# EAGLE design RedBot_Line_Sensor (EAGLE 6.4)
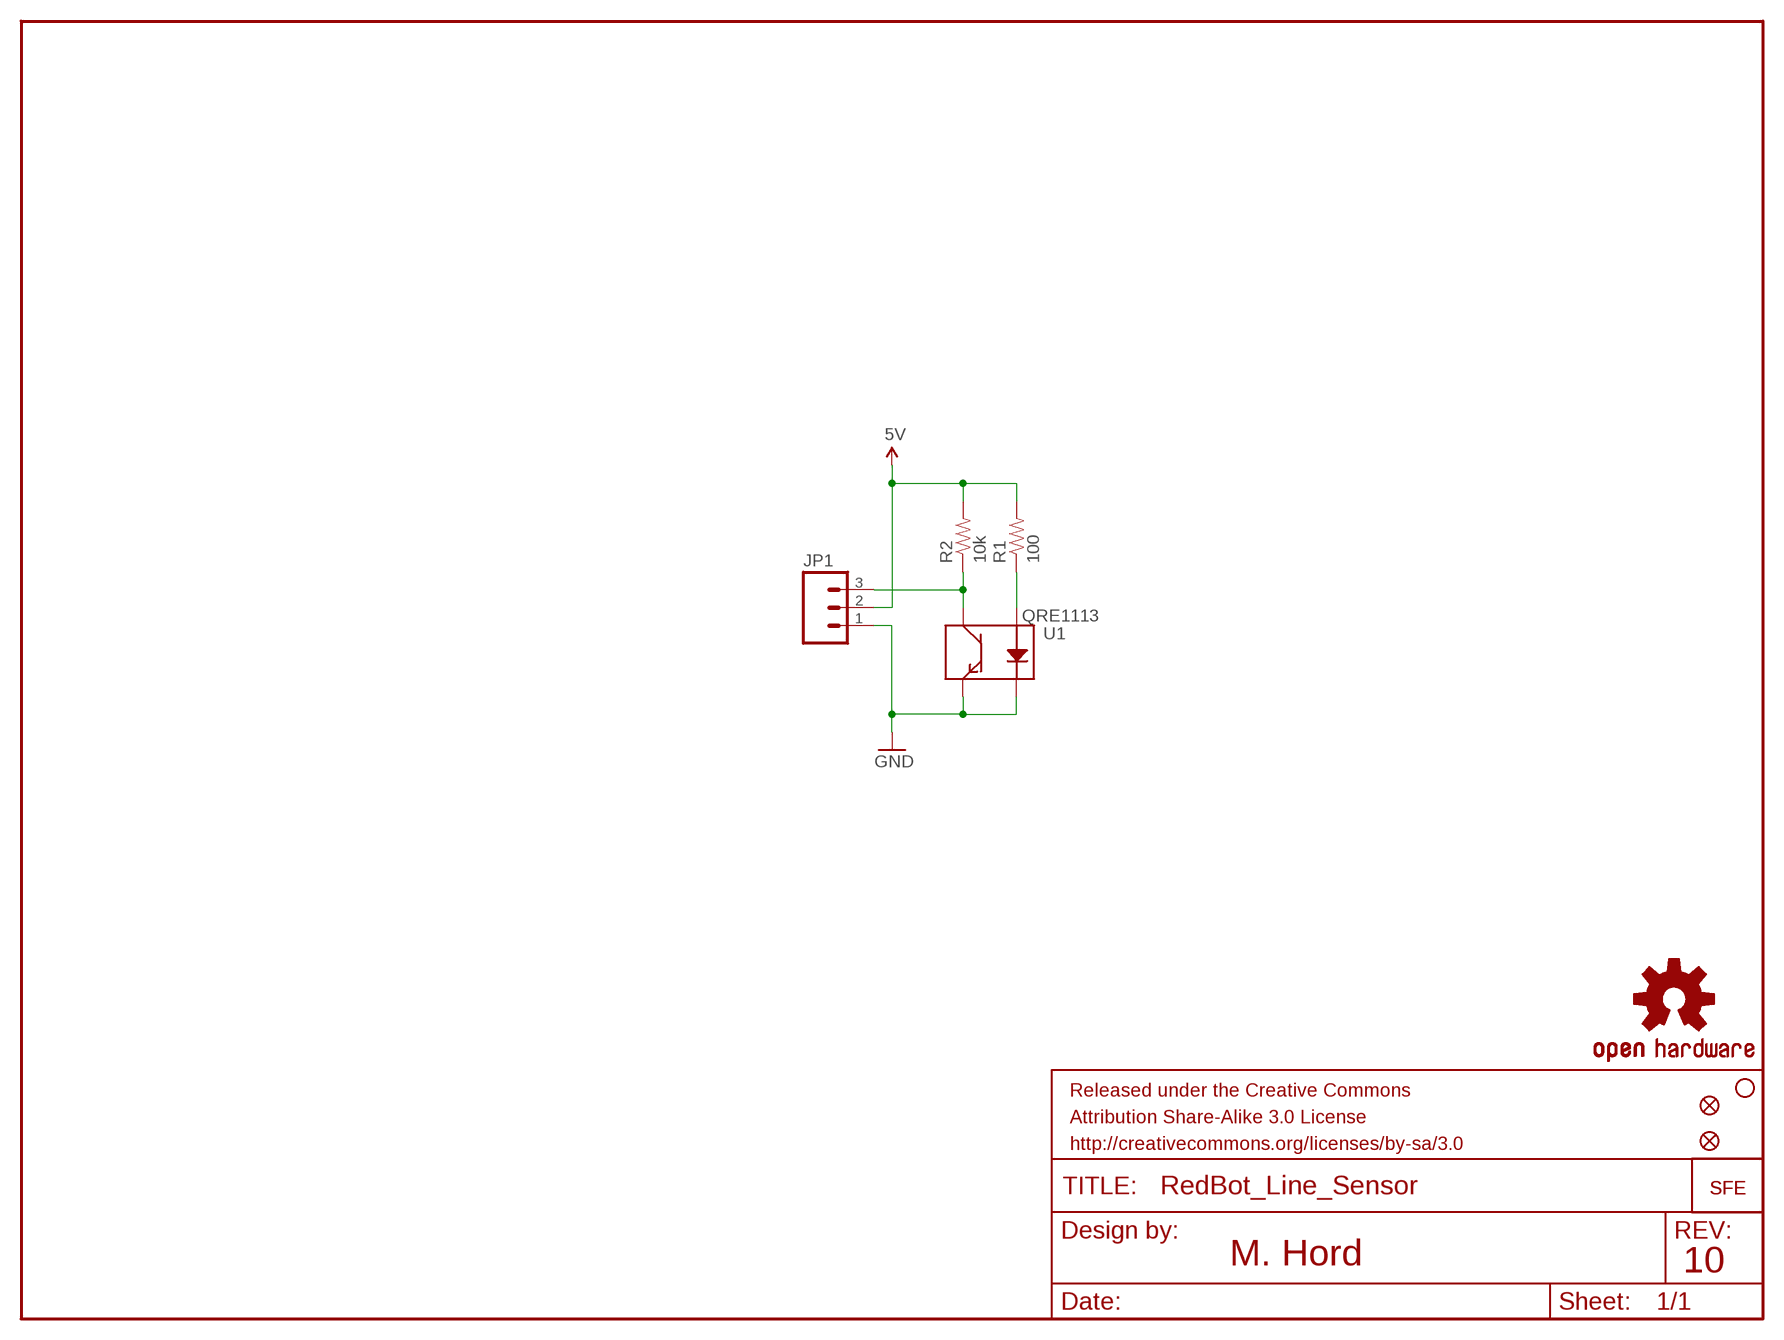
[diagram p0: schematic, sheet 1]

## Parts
FID1  FIDUCIALUFIDUCIAL  [MICRO-FIDUCIAL]
FID2  FIDUCIALUFIDUCIAL  [MICRO-FIDUCIAL]
FRAME1  FRAME-LETTER  [CREATIVE_COMMONS]
JP1  M03SMD_RA_MALE  [1X03_SMD_RA_MALE]
LOGO1  LOGO-SFESK  [SFE-LOGO-FLAME]
LOGO2  OSHW-LOGOS  [OSHW-LOGO-S]
LOGO3  LOGO-SFESK  [SFE-LOGO-FLAME]
R1  100  100-1%  [0402-RES]
R2  10k  10KOHM1/10W1%(0603)  [0402-RES]
STANDOFF1  STAND-OFF  [STAND-OFF]
U1  QRE1113  [QRE1113]

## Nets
5V: JP1.2 R1.2 R2.2
GND: JP1.1 U1.2(K) U1.4(E)
N$1: R1.1 U1.1(A)
N$2: JP1.3 R2.1 U1.3(C)

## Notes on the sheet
- M. Hord | 10

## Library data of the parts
FID1 FID2 = SparkFun-Aesthetics:FIDUCIAL: Fiducial Alignment Points
FRAME1 = SparkFun-Aesthetics:FRAME-LETTER: Schematic Frame
JP1 = SparkFun-Connectors:M03: Header 3 Standard 3-pin 0.1" header. Use with straight break away headers (SKU : PRT-00116), right angle break away headers (PRT-00553), swiss pins (PRT-00743), machine pins (PRT-00117), and female headers (PRT-00115). Molex polarized connector foot print use with SKU : PRT-08232 with associated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; PROD_ID: CONN-10925
LOGO1 LOGO3 = SparkFun-Aesthetics:LOGO-SFE: Spark Fun Electronics PCB Logo
LOGO2 = SparkFun-Aesthetics:OSHW-LOGO: Open Source Hardware Logo This logo indicates the piece of hardware it is found on incorporates a OSHW license and/or adheres to the definition of open source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
R1 = SparkFun-Resistors:100-1%: 100-ohm SMT; PROD_ID: RES-07863
R2 = SparkFun-Resistors:10KOHM1/10W1%(0603): RES-00824; PROD_ID: RES-00824
STANDOFF1 = SparkFun-Electromechanical:STAND-OFF: #4 Stand Off
U1 = SparkFun-Sensors:QRE1113: Reflective object sensor; PROD_ID: IC-09357

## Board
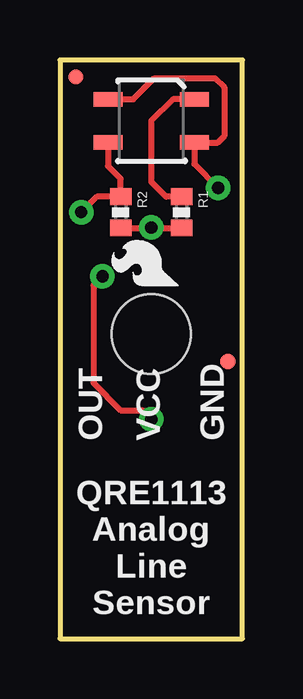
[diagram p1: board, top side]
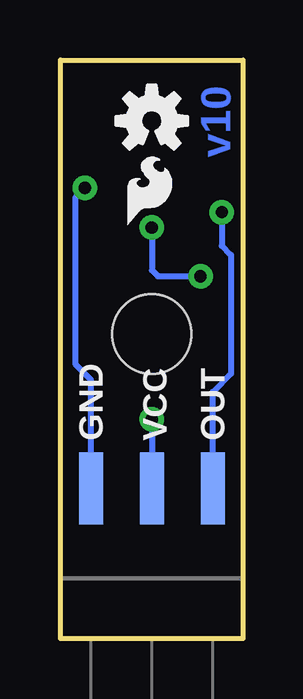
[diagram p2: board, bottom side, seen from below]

Size 7.62 x 24.13 mm. Coordinates in mm from the lower left corner, seen from the top.
Outline: 0,0 7.62,0 7.62,24.13 0,24.13 0,0
Copper layers (1*16): Top 0.035mm / dielectric 1.5mm / Bottom 0.035mm
Design rules "Sparkfun": minimum track width 8mil, minimum drill 20mil, track to track 8mil, track to pad 8mil, pad to pad 8mil, via to via 8mil, smd to smd 8mil, copper to edge 8mil, drill to drill 8mil, minimum pad ring 12mil, minimum via ring 10mil, stop-mask expansion 4mil, vias tented up to drill 20mil, thermal gap 10mil

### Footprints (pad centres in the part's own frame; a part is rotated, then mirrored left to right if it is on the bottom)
MICRO-FIDUCIAL = smd 0.635 x 0.635: 1 0,0
1X03_SMD_RA_MALE = smd 1 x 3: 1 -2.54,5; 2 0,5; 3 2.54,5
0402-RES = smd 0.7 x 0.9: 1 -0.65,0; 2 0.65,0
STAND-OFF = hole 3.302: 0,0
QRE1113 = smd 1.2 x 0.6: 1 -1.8,-0.9; 2 1.8,-0.9; 3 1.8,0.9; 4 -1.8,0.9

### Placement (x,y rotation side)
FID1  7.01,11.56 0 top
FID2  0.66,23.42 0 top
FRAME1  not placed on the board
JP1  3.81,1.27 0 bottom
LOGO1  4.95,14.73 90 top
LOGO2  3.81,21.59 0 bottom
LOGO3  4.83,17.27 0 bottom
R1  5.08,17.78 270 top
R2  2.54,17.78 270 top
STANDOFF1  3.81,12.7 0 top
U1  3.81,21.59 180 top

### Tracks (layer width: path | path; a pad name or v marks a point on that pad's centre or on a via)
5V  (via drill 0.51)
  Top 0.254: R2.2 3.82,17.13 | 3.82,17.13 R1.2 | 3.82,17.13 v3.81,17.14 | v1.78,15.11 1.4,14.73 1.4,10.67 2.54,9.53 3.43,9.53 v3.81,9.14
  Bottom 0.254: v3.81,17.14 3.81,15.37 3.56,15.11 v1.78,15.11 | v3.81,9.14 JP1.2
GND  (via drill 0.51)
  Top 0.254: U1.2 3.06,22.49 3.94,23.37 6.48,23.37 6.86,22.99 6.86,20.95 6.59,20.69 U1.4 5.61,19.79 v6.6,18.8
  Bottom 0.254: JP1.1 6.35,10.79 6.99,11.43 6.99,18.41 v6.6,18.8
N$1
  Top 0.254: U1.1 4.71,22.49 3.81,21.59 3.81,19.05 4.43,18.43 R1.1
N$2  (via drill 0.51)
  Top 0.254: U1.3 2.01,19.71 2.54,19.18 R2.1 1.54,18.43 v0.89,17.78
  Bottom 0.254: JP1.3 1.27,10.29 0.51,11.05 0.51,16 0.89,16.38 v0.89,17.78

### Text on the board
Bottom: v10
tPlace: OUT | VCC | GND | QRE1113 / Analog / Line / Sensor
bPlace: OUT | VCC | GND
tNames: M.Hord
